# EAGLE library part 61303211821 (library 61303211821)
Wurth Elektronik 6130 Series, Series Number 613032, 2.54mm Pitch 32 Way 1 Row Straight PCB Header, Solder Termination Source: Datasheet
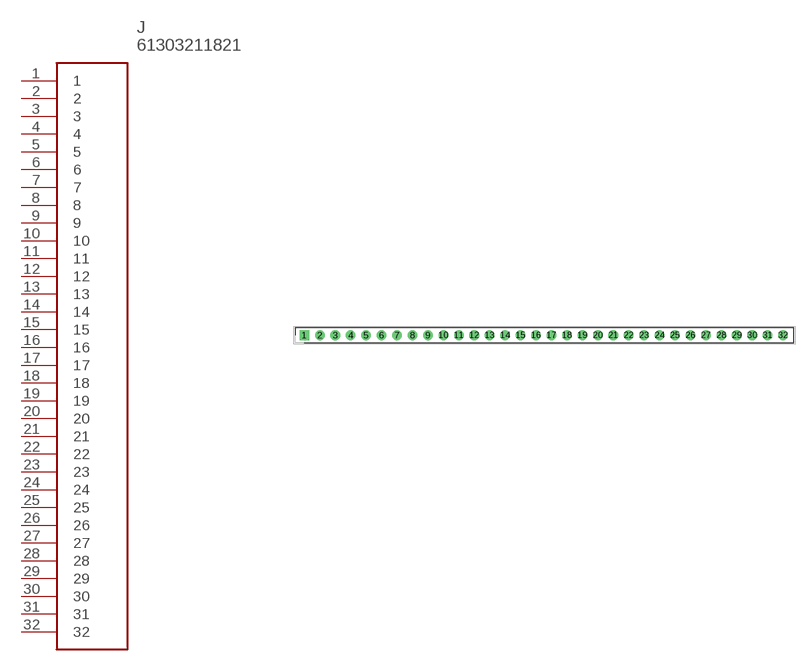
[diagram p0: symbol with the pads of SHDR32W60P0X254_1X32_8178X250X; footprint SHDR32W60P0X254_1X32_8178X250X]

Designator prefix J

## 61303211821 (Description: Wurth Elektronik 6130 Series, Series Number 613032, 2.54mm Pitch 32 Way 1 Row Straight PCB Header, Solder Termination; Height: 8.5mm; Manufacturer_Name: Wurth Elektronik; Manufacturer_Part_Number: 61303211821; Mouser_Part_Number: 710-61303211821; Mouser_Price-Stock: https://www.mouser.co.uk/ProductDetail/Wurth-Elektronik/61303211821?qs=ZtY9WdtwX55M%2FH%2FSrHZ9xA%3D%3D)  [SHDR32W60P0X254_1X32_8178X250X]
1  1
2  2
3  3
4  4
5  5
6  6
7  7
8  8
9  9
10  10
11  11
12  12
13  13
14  14
15  15
16  16
17  17
18  18
19  19
20  20
21  21
22  22
23  23
24  24
25  25
26  26
27  27
28  28
29  29
30  30
31  31
32  32

## Footprint SHDR32W60P0X254_1X32_8178X250X (pad centres in mm)
61303211821
drill 1.05 pad 1.575 square: 1 0,0
drill 1.05 pad 1.575: 2 2.54,0; 3 5.08,0; 4 7.62,0; 5 10.16,0; 6 12.7,0; 7 15.24,0; 8 17.78,0; 9 20.32,0; 10 22.86,0; 11 25.4,0; 12 27.94,0; 13 30.48,0; 14 33.02,0; 15 35.56,0; 16 38.1,0; 17 40.64,0; 18 43.18,0; 19 45.72,0; 20 48.26,0; 21 50.8,0; 22 53.34,0; 23 55.88,0; 24 58.42,0; 25 60.96,0; 26 63.5,0; 27 66.04,0; 28 68.58,0; 29 71.12,0; 30 73.66,0; 31 76.2,0; 32 78.74,0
